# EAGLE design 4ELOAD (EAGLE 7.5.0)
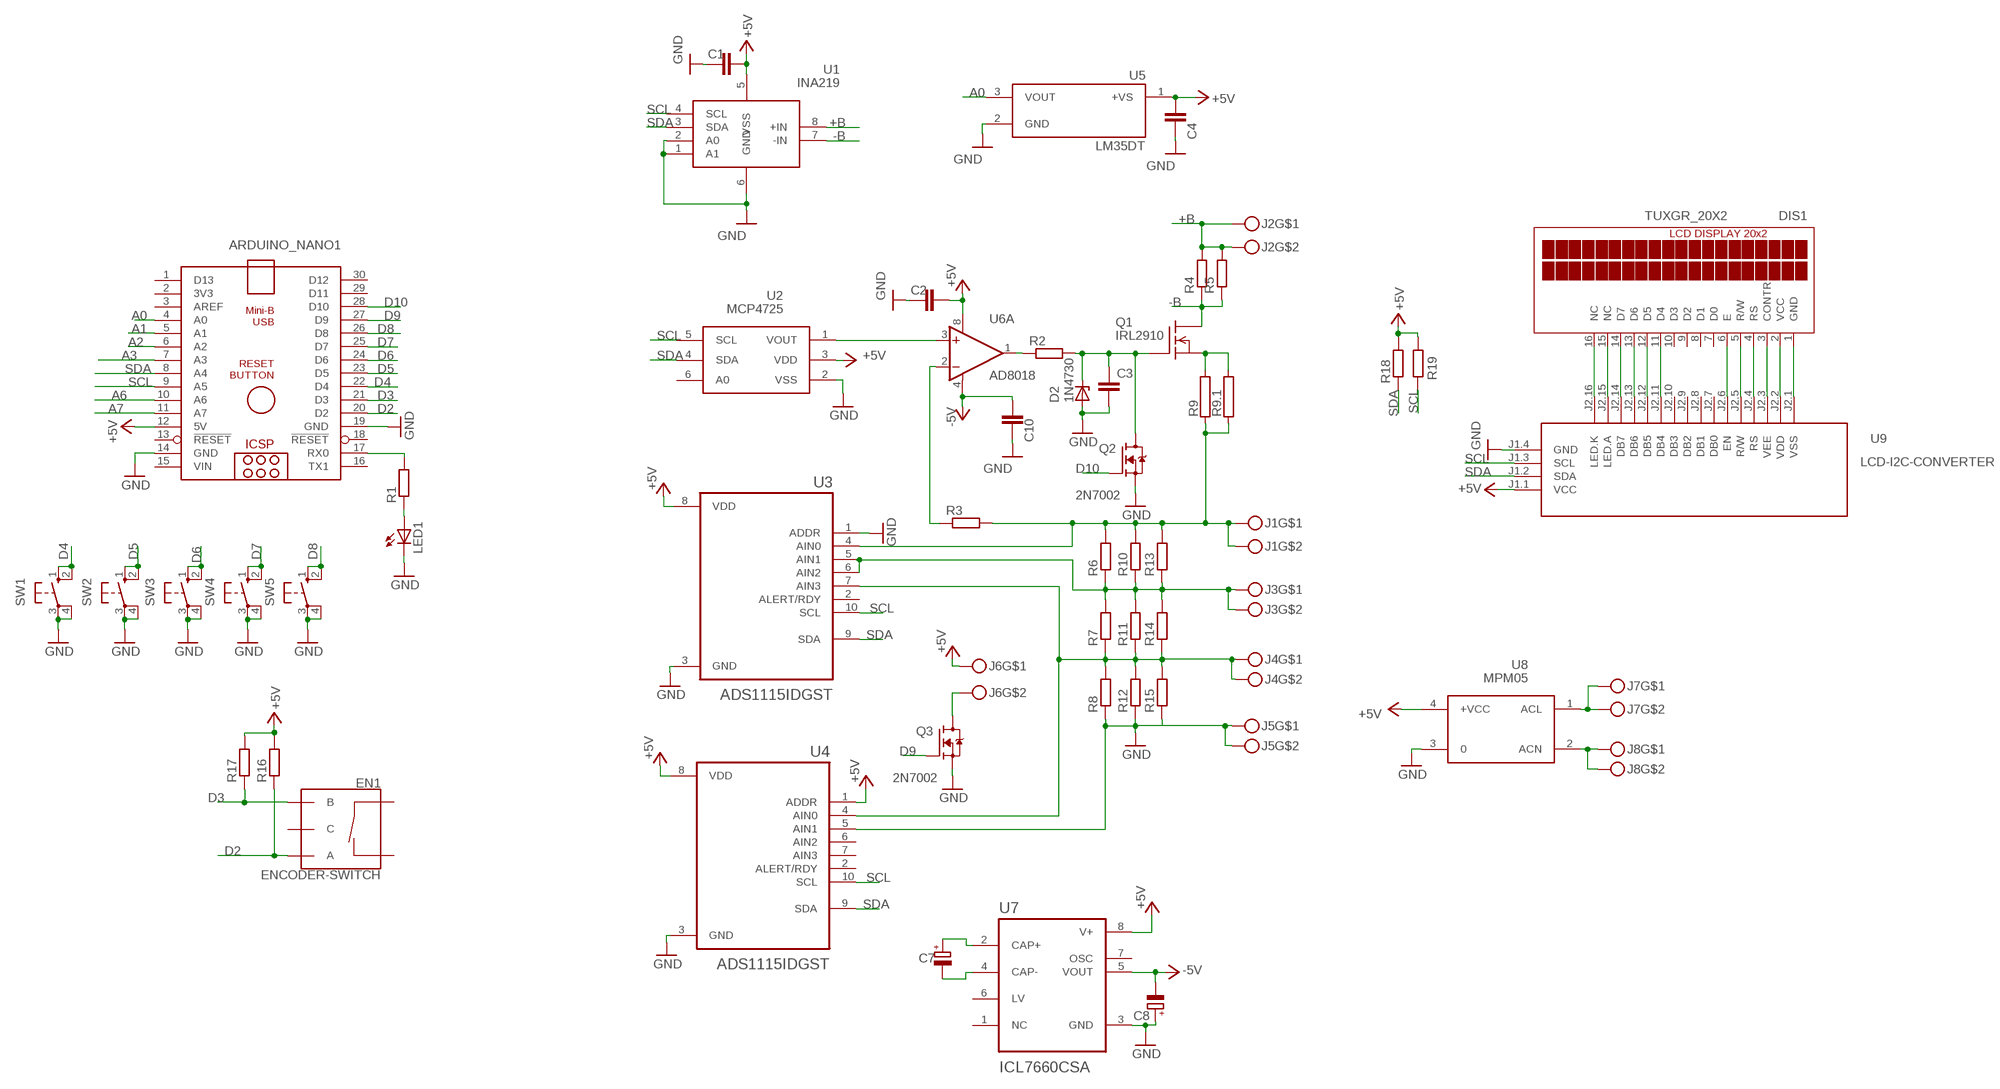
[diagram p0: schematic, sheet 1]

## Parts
ARDUINO_NANO1  ARDUINO_NANO  [ARDUINO_NANO]
C1  C-EUC1206  [C1206]
C2  C-EUC1206  [C1206]
C3  C-EUC1206  [C1206]
C4  C-EUC1206  [C1206]
C7  CPOL-EUSMCB  [SMC_B]
C8  CPOL-EUSMCB  [SMC_B]
C10  C-EUC1206  [C1206]
D2  1N4730  BZX85  [DO41Z10]
DIS1  TUXGR_20X2  [TUXGR_20X2]
EN1  ENCODER-SWITCH  [ROTARY_ENC_PLAIN]
J1  MKDSN1,5-2-5,08  [MKDSN1,5-2-5,08]
J2  MKDSN1,5-2-5,08  [MKDSN1,5-2-5,08]
J3  MKDSN1,5-2-5,08  [MKDSN1,5-2-5,08]
J4  MKDSN1,5-2-5,08  [MKDSN1,5-2-5,08]
J5  MKDSN1,5-2-5,08  [MKDSN1,5-2-5,08]
J6  MKDSN1,5-2-5,08  [MKDSN1,5-2-5,08]
J7  MKDSN1,5-2-5,08  [MKDSN1,5-2-5,08]
J8  MKDSN1,5-2-5,08  [MKDSN1,5-2-5,08]
LED1  LED5MM  [LED5MM]
Q1  IRL2910  BUZ21  [TO220]
Q2  2N7002  [SOT95P240X111-3N]
Q3  2N7002  [SOT95P240X111-3N]
R1  R-EU_R1206  [R1206]
R2  R-EU_R1206  [R1206]
R3  R-EU_R1206  [R1206]
R4  R-EU_R2512  [R2512]
R5  R-EU_R2512  [R2512]
R6  R-EU_R2512  [R2512]
R7  R-EU_R2512  [R2512]
R8  R-EU_R2512  [R2512]
R9  RCA5100  [CA5100]
R9.1  RCA5100  [CA5100]
R10  R-EU_R2512  [R2512]
R11  R-EU_R2512  [R2512]
R12  R-EU_R2512  [R2512]
R13  R-EU_R2512  [R2512]
R14  R-EU_R2512  [R2512]
R15  R-EU_R2512  [R2512]
R16  R-EU_R1206  [R1206]
R17  R-EU_R1206  [R1206]
R18  R-EU_R1206  [R1206]
R19  R-EU_R1206  [R1206]
SW1  10-XX  [B3F-10XX]
SW2  10-XX  [B3F-10XX]
SW3  10-XX  [B3F-10XX]
SW4  10-XX  [B3F-10XX]
SW5  10-XX  [B3F-10XX]
U1  INA219  [SO08]
U2  MCP4725  [SOT23-6]
U3  ADS1115IDGST  [SOP50P490X110-10N]
U4  ADS1115IDGST  [SOP50P490X110-10N]
U5  LM35DT  [TO254P1016X457X1955-3]
U6  AD8018  OPA2650U  [SO08]
U7  ICL7660CSA  [SOIC127P600X175-8N]
U8  MPM05  [MPM05]
U9  LCD-I2C-CONVERTER  [LCD-I2C-CONVERTER]

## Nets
+5V: ARDUINO_NANO1.12(5V) C1.1 C2.1 C4.1 DIS1.2(VCC) J6.1 R16.2 R17.2 R18.2 R19.2 U1.5(VSS) U2.3(VDD) U3.8(VDD) U4.1(ADDR) U4.8(VDD) U5.1(+VS) U6.8(A:V+) U7.8(V+) U8.4(+VCC) U9.J1.1(VCC) U9.J2.2(VDD)
+B: J2.1 J2.2 R4.2 R5.2 U1.8(+IN)
-5V: C8.- C10.1 U6.4(A:V-) U7.5(VOUT)
-B: Q1.2(D) R4.1 R5.1 U1.7(-IN)
A0: ARDUINO_NANO1.4(A0) U5.3(VOUT)
A1: ARDUINO_NANO1.5(A1)
A2: ARDUINO_NANO1.6(A2)
A3: ARDUINO_NANO1.7(A3)
A6: ARDUINO_NANO1.10(A6)
A7: ARDUINO_NANO1.11(A7)
D2: ARDUINO_NANO1.20(D2) EN1.A R16.1
D3: ARDUINO_NANO1.21(D3) EN1.B R17.1
D4: ARDUINO_NANO1.22(D4) SW1.1(S) SW1.2(S1)
D5: ARDUINO_NANO1.23(D5) SW2.1(S) SW2.2(S1)
D6: ARDUINO_NANO1.24(D6) SW3.1(S) SW3.2(S1)
D7: ARDUINO_NANO1.25(D7) SW4.1(S) SW4.2(S1)
D8: ARDUINO_NANO1.26(D8) SW5.1(S) SW5.2(S1)
D9: ARDUINO_NANO1.27(D9) Q3.1(G)
D10: ARDUINO_NANO1.28(D10) Q2.1(G)
GND: ARDUINO_NANO1.14(GND) ARDUINO_NANO1.19(GND) C1.2 C2.2 C3.2 C4.2 C8.+ C10.2 D2.A DIS1.1(GND) J5.1 J5.2 LED1.K(C) Q2.2(S) Q3.2(S) R8.1 R12.1 R15.1 SW1.3(P) SW1.4(P1) SW2.3(P) SW2.4(P1) SW3.3(P) SW3.4(P1) SW4.3(P) SW4.4(P1) SW5.3(P) SW5.4(P1) U1.1(A1) U1.2(A0) U1.6(GND) U2.2(VSS) U3.1(ADDR) U3.3(GND) U4.3(GND) U4.5(AIN1) U5.2(GND) U7.3(GND) U8.3 U9.J1.4(GND) U9.J2.1(VSS)
N$1: U2.1(VOUT) U6.3(A:+IN)
N$2: C3.1 D2.C Q1.1(G) Q2.3(D) R2.2
N$3: R2.1 U6.1(A:OUT)
N$4: Q1.3(S) R9.1.2 R9.2
N$5: R3.1 U6.2(A:-IN)
N$6: J1.1 J1.2 R3.2 R6.2 R9.1 R9.1.1 R10.2 R13.2 U3.4(AIN0)
N$7: ARDUINO_NANO1.17(RX0) R1.2
N$8: LED1.A R1.1
N$9: J3.1 J3.2 R6.1 R7.2 R10.1 R11.2 R13.1 R14.2 U3.5(AIN1) U3.6(AIN2)
N$10: J4.1 J4.2 R7.1 R8.2 R11.1 R12.2 R14.1 R15.2 U3.7(AIN3) U4.4(AIN0)
N$11: C7.+ U7.2(CAP+)
N$12: C7.- U7.4(CAP-)
N$13: J6.2 Q3.3(D)
N$15: J7.1 J7.2 U8.1(ACL)
N$16: J8.1 J8.2 U8.2(ACN)
N$31: DIS1.3(CONTR) U9.J2.3(VEE)
N$32: DIS1.4(RS) U9.J2.4(RS)
N$33: DIS1.5(R/W) U9.J2.5(R/W)
N$34: DIS1.6(E) U9.J2.6(EN)
N$35: DIS1.14(D7) U9.J2.14(DB7)
N$36: DIS1.13(D6) U9.J2.13(DB6)
N$37: DIS1.12(D5) U9.J2.12(DB5)
N$38: DIS1.11(D4) U9.J2.11(DB4)
N$39: DIS1.16(NC) U9.J2.16(LED.K)
N$40: DIS1.15(NC) U9.J2.15(LED.A)
SCL: ARDUINO_NANO1.9(A5) R19.1 U1.4(SCL) U2.5(SCL) U3.10(SCL) U4.10(SCL) U9.J1.3(SCL)
SDA: ARDUINO_NANO1.8(A4) R18.1 U1.3(SDA) U2.4(SDA) U3.9(SDA) U4.9(SDA) U9.J1.2(SDA)
Unconnected: ARDUINO_NANO1.1(D13) ARDUINO_NANO1.2(3V3) ARDUINO_NANO1.3(AREF) ARDUINO_NANO1.13(!RESET) ARDUINO_NANO1.16(TX1) ARDUINO_NANO1.18(!RESET) ARDUINO_NANO1.29(D11) ARDUINO_NANO1.30(D12) DIS1.7(D0) DIS1.8(D1) DIS1.9(D2) DIS1.10(D3) EN1.C EN1.SW+ EN1.SW- U2.6(A0) U3.2(ALERT/RDY) U4.2(ALERT/RDY) U4.6(AIN2) U4.7(AIN3) U6.5(B:+IN) U6.6(B:-IN) U6.7(B:OUT) U7.1(NC) U7.6(LV) U7.7(OSC) U9.J2.7(DB0) U9.J2.8(DB1) U9.J2.9(DB2) U9.J2.10(DB3)

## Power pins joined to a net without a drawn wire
VIN: ARDUINO_NANO1.15(VIN)

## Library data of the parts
ARDUINO_NANO1 = ArduinoNanoV30:ARDUINO_NANO: Arduino Nano V3.0 Overview: The Arduino Nano is a small, complete, and breadboard-friendly board based on the ATmega328 (Arduino Nano 3.x) or ATmega168 (Arduino Nano 2.x). It has more or less the same functionality of the Arduino Duemilanove, but in a different package. It lacks only a DC power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
C1-C4 C10 = rcl:C-EU: CAPACITOR, European symbol
C7 C8 = rcl:CPOL-EU: POLARIZED CAPACITOR, European symbol
D2 = diode:BZX85: Z DIODE
DIS1 = display-lcd:TUXGR_20X2: Tuxgraphics LCD display 20x2 characters reflective, without background light Source: tuxgr_20x2.pdf; OC_FARNELL: unknown; OC_NEWARK: unknown
EN1 = SparkFun-Switches:ENCODER-SWITCH: Rotary Encoder w/ Select Switch Encoders rotate similarly to potentiometers, but they’re different from potentiometers in that an encoder has full rotation without limits. They output gray code so that you can tell how much and in which direction the encoder has been turned. This encoder includes a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; SF_SKU: COM-09117
J1-J8 = con-phoenix-508:MKDSN1,5-2-5,08
LED1 = led:LED: LED
Q1 = transistor-fet:BUZ21: N-Channel Enhancement MOSFET 100V; 19A; 0,1Ohm
Q2 Q3 = 2N7002:2N7002: Check availability; AVAILABILITY: In Stock; CHECK_PRICES: https://www.snapeda.com/parts/2N7002/Onsemi/view-part/?ref=eda; DESCRIPTION: Mosfet Array 2 N-Channel (Dual) 60V 300mA 500mW Surface Mount PG-SOT363-6; MF: onsemi; MP: 2N7002; PACKAGE: SOT-23-3 ON Semiconductor; PRICE: None; SNAPEDA_LINK: https://www.snapeda.com/parts/2N7002/Onsemi/view-part/?ref=snap
R1-R8 R10-R19 = rcl:R-EU_: RESISTOR, European symbol
R9 R9.1 = resistor-power:R: Power Resitor; OC_FARNELL: unknown; OC_NEWARK: unknown
SW1-SW5 = switch-omron:10-XX: OMRON SWITCH; MPN: B3F-1000; OC_FARNELL: 176432; OC_NEWARK: 36M3542
U1 = burr-brown:INA219: Bidirectional Current/Power Monitor With I2C Interface
U2 = linear:MCP4725
U3 U4 = ADS1115IDGST:ADS1115IDGST: Check availability; AVAILABILITY: In Stock; CHECK_PRICES: https://www.snapeda.com/parts/ADS1115IDGST/Texas+Instruments/view-part/?ref=eda; DESCRIPTION: 16-bit, 860-SPS, 4-channel, delta-sigma ADC with PGA, oscillator, VREF, comparator and I2C; MF: Texas Instruments; MP: ADS1115IDGST; PACKAGE: VSSOP-10 Texas Instruments; PRICE: None; SNAPEDA_LINK: https://www.snapeda.com/parts/ADS1115IDGST/Texas+Instruments/view-part/?ref=snap
U5 = LM35DT-H:LM35DT: Check availability; AVAILABILITY: In Stock; CHECK_PRICES: https://www.snapeda.com/parts/LM35DT/Texas+Instruments/view-part/?ref=eda; DESCRIPTION: ±0.5°C 4V-30V, Temperature sensor with analog output 3-TO-220 0 to 100; MF: Texas Instruments; MP: LM35DT; PACKAGE: TO-220-3 Texas Instruments; PRICE: None; SNAPEDA_LINK: https://www.snapeda.com/parts/LM35DT/Texas+Instruments/view-part/?ref=snap
U6 = burr-brown:OPA2650: Dual Wideband, Low Power Voltage Feedback Operational Amplifier; MF: ALTERA CORPORATION; MPN: AD8056ARMZ; OC_FARNELL: 1424046; OC_NEWARK: 59K6306
U7 = ICL7660CSA:ICL7660CSA: Check availability; AVAILABILITY: In Stock; CHECK_PRICES: https://www.snapeda.com/parts/ICL7660CSA/Analog+Devices/view-part/?ref=eda; DESCRIPTION: Charge Pump Switching Regulator IC Positive or Negative Fixed -Vin, nVin, Vin/2 1 Output 20mA 8-SOIC (0.154, 3.90mm Width); MF: Analog Devices; MP: ICL7660CSA; PACKAGE: SOIC-8 Maxim; PRICE: None; SNAPEDA_LINK: https://www.snapeda.com/parts/ICL7660CSA/Analog+Devices/view-part/?ref=snap
U8 = acdc:MPM05: AC DC Converter 5W
U9 = diy-modules:LCD-I2C-CONVERTER: I2C Bus to 4-Bit Parallel LCD Interface with LED backlight driver

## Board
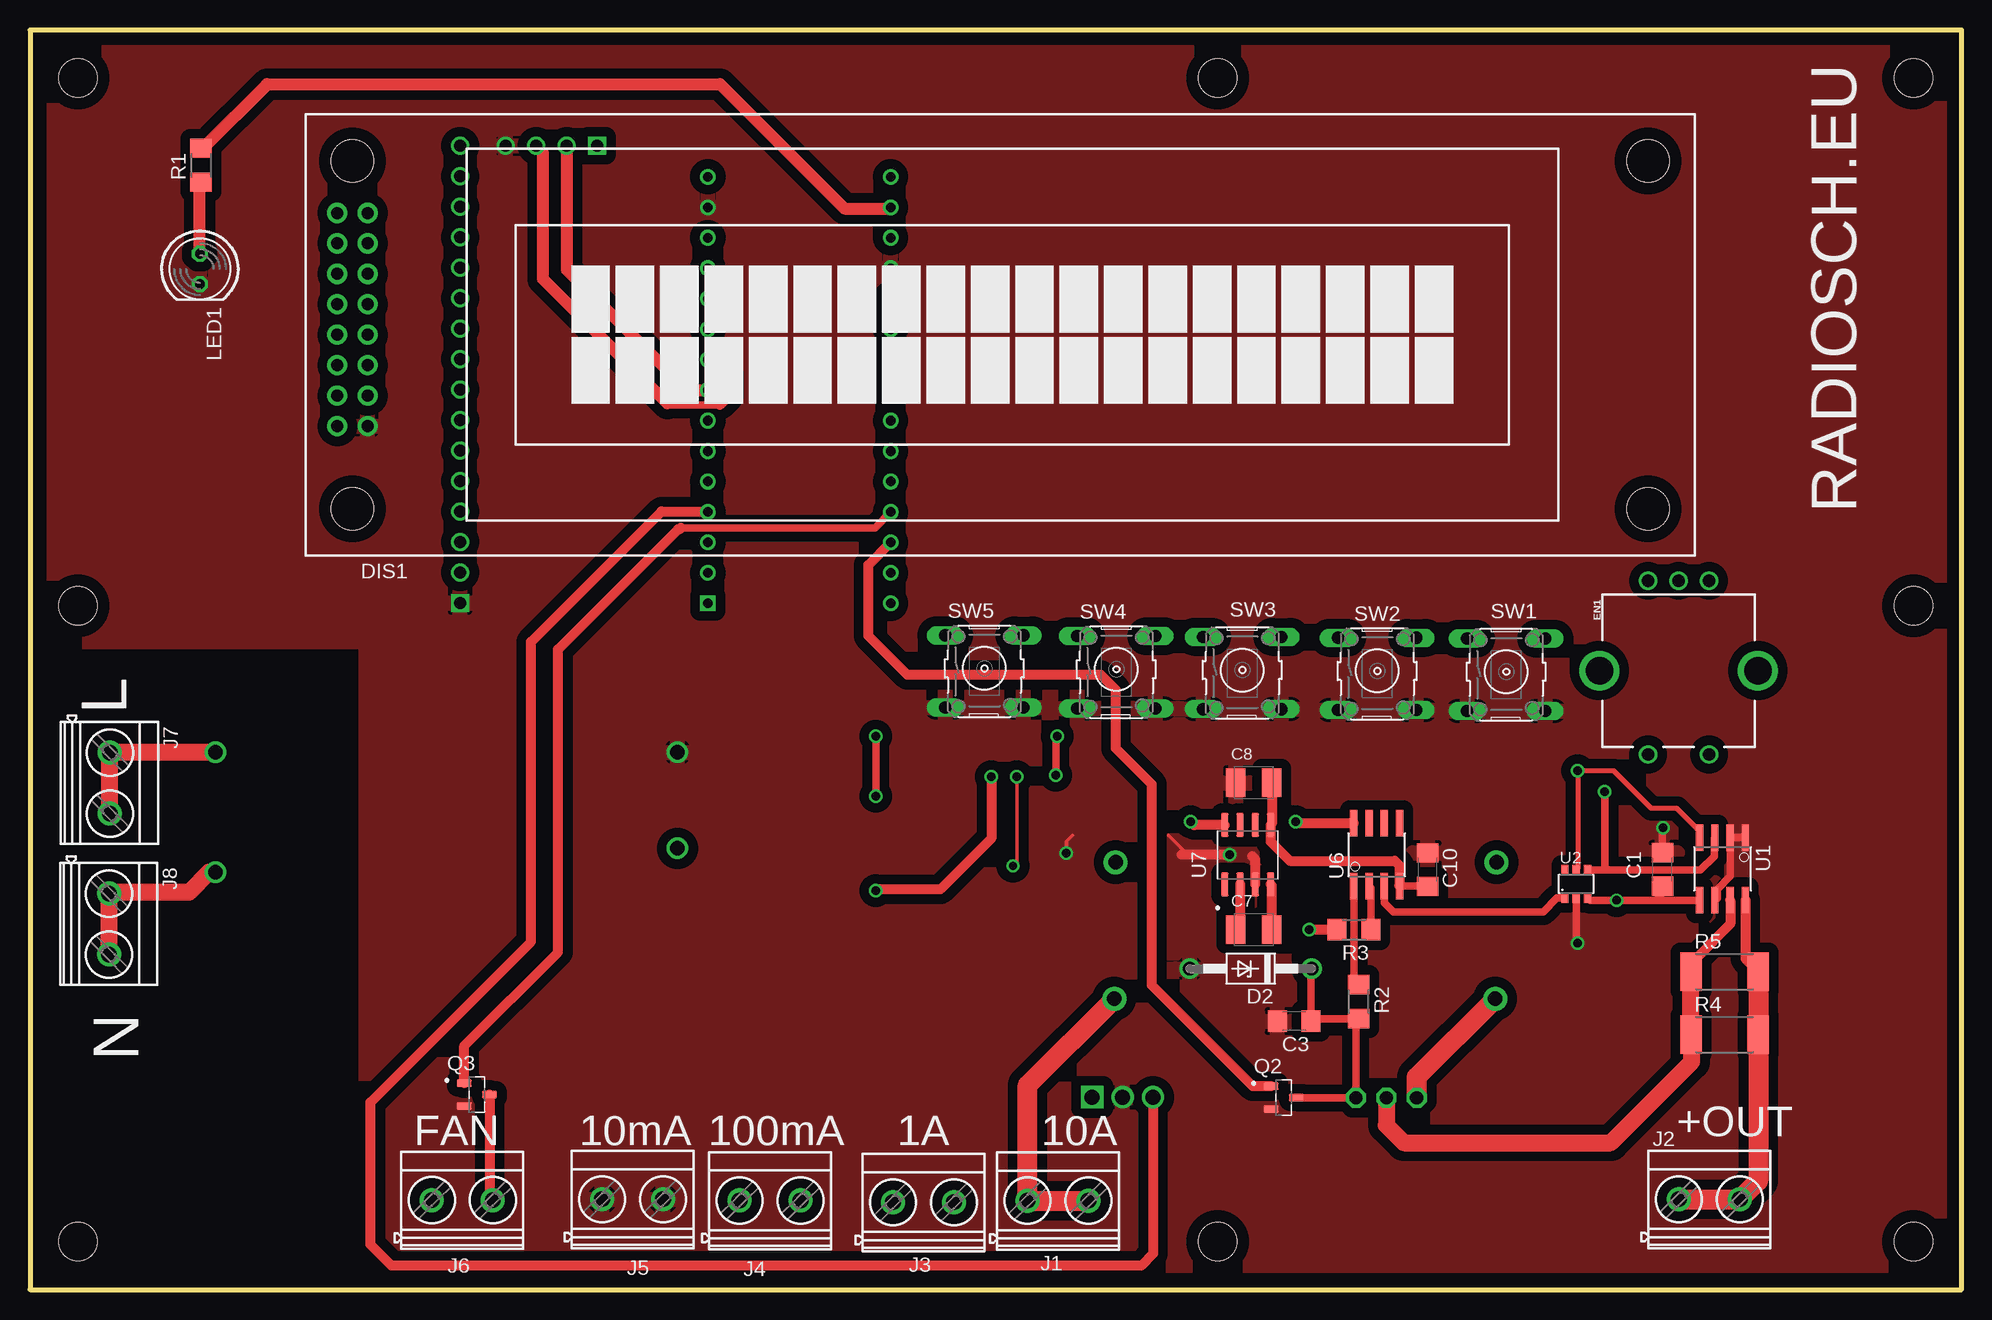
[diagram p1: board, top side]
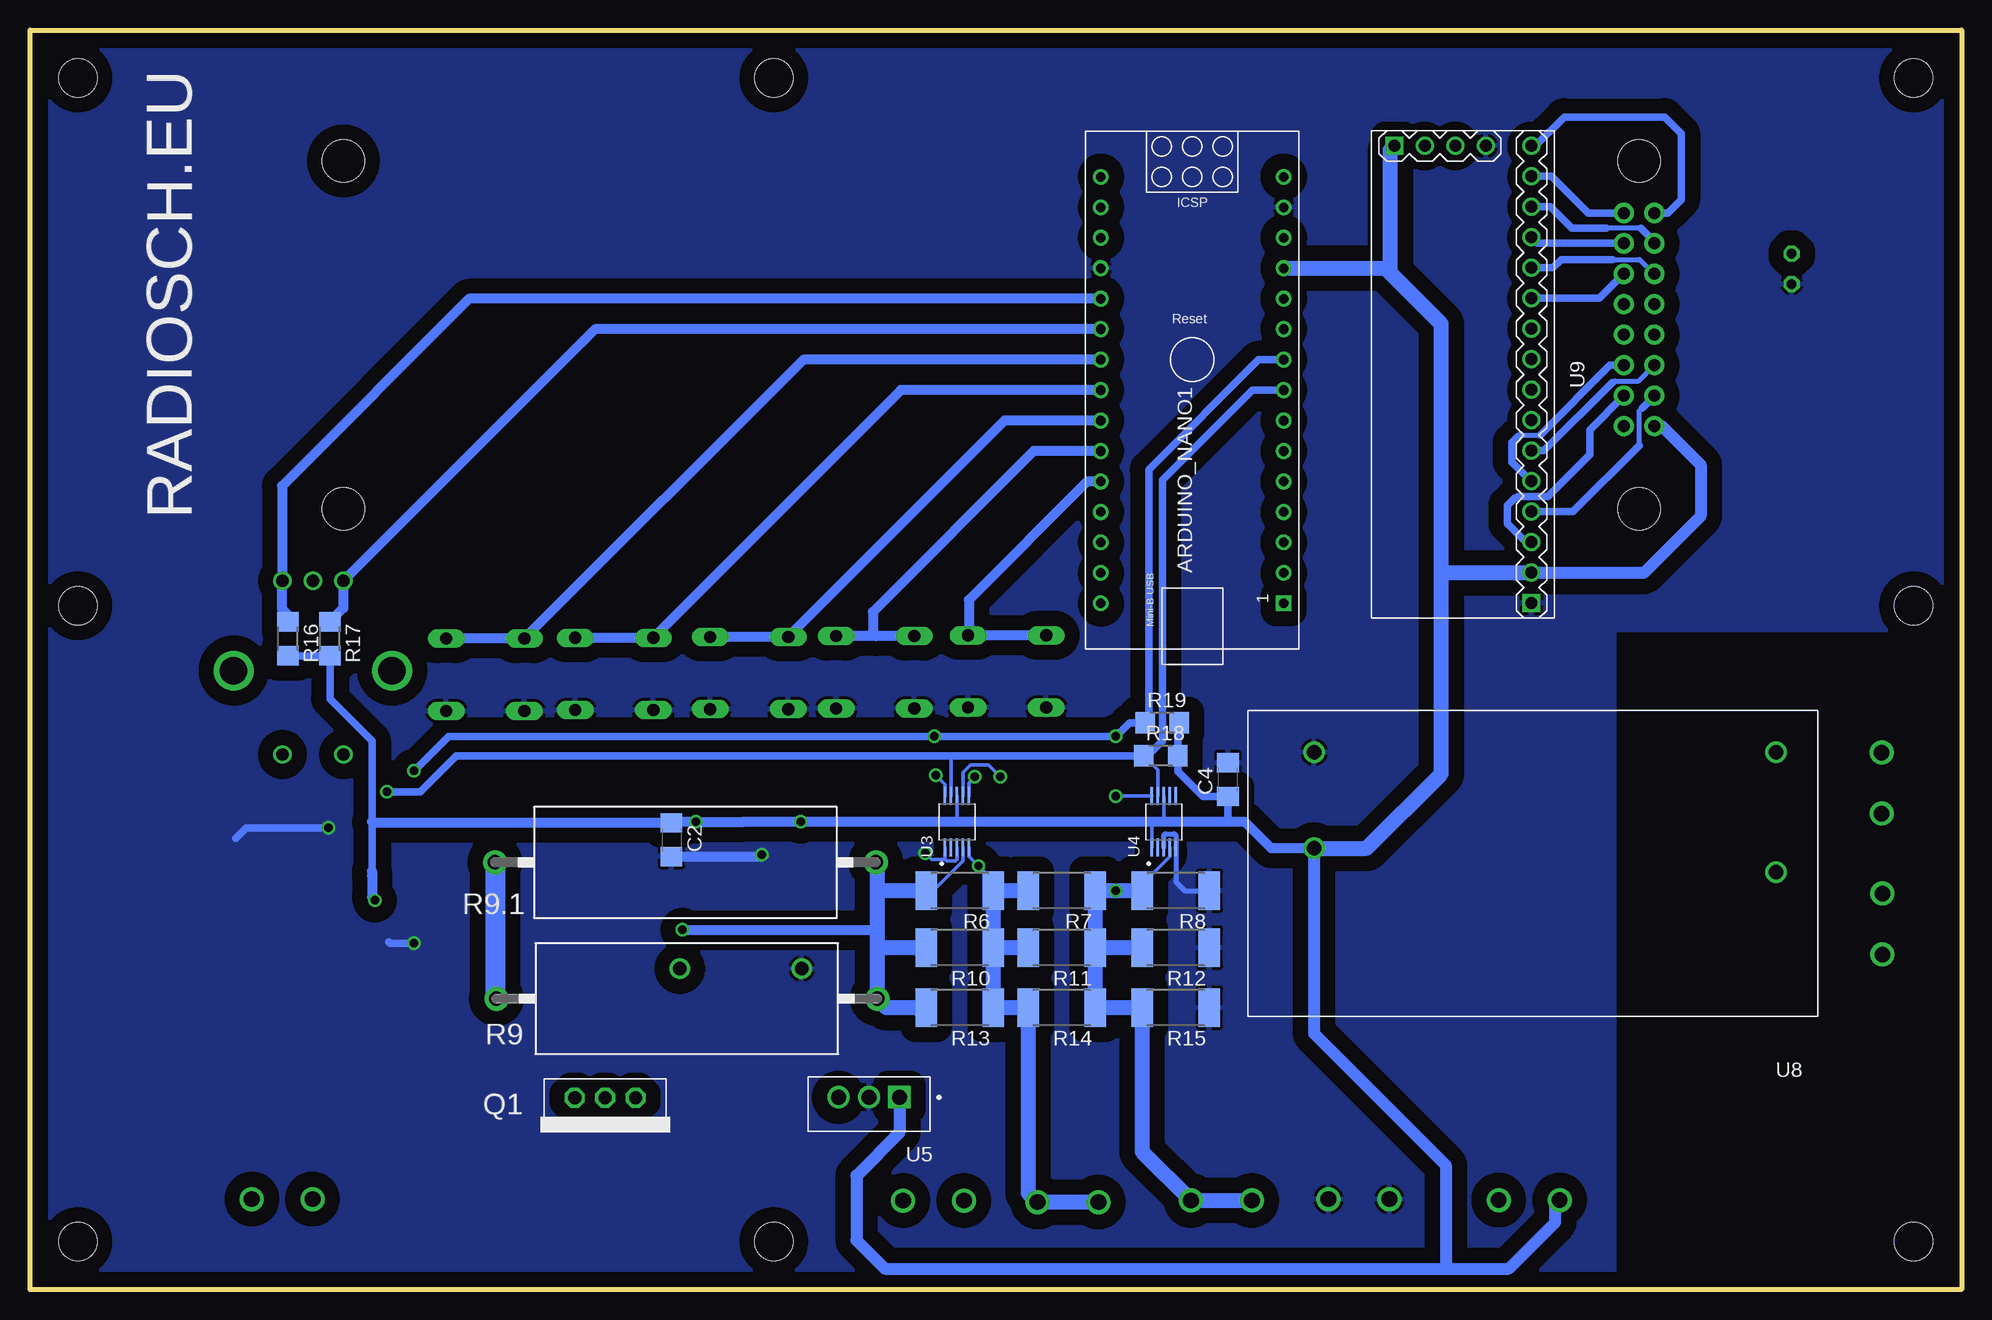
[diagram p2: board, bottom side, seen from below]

Size 161 x 105 mm. Coordinates in mm from the lower left corner, seen from the top.
Outline: 0,0 161,0 161,105 0,105 0,0
Copper layers (1*16): Top 0.035mm / dielectric 1.5mm / Bottom 0.035mm
Design rules "default *": minimum track width 10mil, minimum drill 24mil, track to track 4mil, track to pad 4mil, pad to pad 4mil, via to via 8mil, smd to smd 4mil, copper to edge 40mil, drill to drill 8mil, minimum pad ring 10mil, minimum via ring 8mil, stop-mask expansion 4mil, vias tented up to drill 0mil, thermal gap 10mil
Holes 3.2 mm at 4,4 99,4 157,4 4,57 157,57 157,101 99,101 4,101

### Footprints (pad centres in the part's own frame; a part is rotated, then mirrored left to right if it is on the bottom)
ARDUINO_NANO = drill 0.8 square: 1 -20.32,-7.62 | drill 0.8: 2 -17.78,-7.62; 3 -15.24,-7.62; 4 -12.7,-7.62; 5 -10.16,-7.62; 6 -7.62,-7.62; 7 -5.08,-7.62; 8 -2.54,-7.62; 9 0,-7.62; 10 2.54,-7.62; 11 5.08,-7.62; 12 7.62,-7.62; 13 10.16,-7.62; 14 12.7,-7.62; 15 15.24,-7.62; 16 15.24,7.62; 17 12.7,7.62; 18 10.16,7.62; 19 7.62,7.62; 20 5.08,7.62; 21 2.54,7.62; 22 0,7.62; 23 -2.54,7.62; 24 -5.08,7.62; 25 -7.62,7.62; 26 -10.16,7.62; 27 -12.7,7.62; 28 -15.24,7.62; 29 -17.78,7.62; 30 -20.32,7.62
C1206 = smd 1.6 x 1.8: 1 -1.4,0; 2 1.4,0
SMC_B = smd 1.6 x 2.4: + -1.5,0; - 1.5,0
DO41Z10 = drill 1.118: A 5.08,0; C -5.08,0
TUXGR_20X2 = drill 1 pad 1.676: 1 -52.73,-7.62; 2 -55.27,-7.62; 3 -52.73,-5.08; 4 -55.27,-5.08; 5 -52.73,-2.54; 6 -55.27,-2.54; 7 -52.73,0; 8 -55.27,0; 9 -52.73,2.54; 10 -55.27,2.54; 11 -52.73,5.08; 12 -55.27,5.08; 13 -52.73,7.62; 14 -55.27,7.62; 15 -52.73,10.16; 16 -55.27,10.16 | hole 3.5: -54,-14.5; 54,-14.5; -54,14.5; 54,14.5
ROTARY_ENC_PLAIN = drill 1.016: A 7.493,-2.54; B 7.493,2.54; C 7.493,0; SW+ -6.985,2.54; SW- -6.985,-2.54 | drill 2.286: P$3 0,6.604; P$4 0,-6.604
MKDSN1,5-2-5,08 = drill 1.3 pad 2: 1 -2.561,0.025; 2 2.519,0.025
LED5MM = drill 0.813 octagon: A -1.27,0; K 1.27,0
TO220 = drill 1.118 octagon: 1 -2.54,0; 2 0,0; 3 2.54,0
SOT95P240X111-3N = smd 1.23 x 0.6: 1 -1.06,0.95; 2 -1.06,-0.95; 3 1.06,0
R1206 = smd 1.6 x 1.803: 1 -1.422,0; 2 1.422,0
R2512 = smd 1.8 x 3.2: 1 -2.8,0; 2 2.8,0
CA5100 = drill 1.2 pad 2: 1 -15.875,0; 2 15.875,0
B3F-10XX = drill 1.016 long: 1 -3.251,2.761; 2 3.251,2.761; 3 -3.251,-3.261; 4 3.251,-3.261
SO08 = smd 0.61 x 2.21: 1 -1.905,-2.616; 2 -0.635,-2.616; 3 0.635,-2.616; 4 1.905,-2.616; 5 1.905,2.616; 6 0.635,2.616; 7 -0.635,2.616; 8 -1.905,2.616
SOT23-6 = smd 0.6 x 0.9: 1 -0.95,-1.15; 2 0,-1.15; 3 0.95,-1.15; 4 0.95,1.15; 5 0,1.15; 6 -0.95,1.15
SOP50P490X110-10N = smd 1.47 x 0.28: 1 -2.15,1; 2 -2.15,0.5; 3 -2.15,0; 4 -2.15,-0.5; 5 -2.15,-1; 6 2.15,-1; 7 2.15,-0.5; 8 2.15,0; 9 2.15,0.5; 10 2.15,1
TO254P1016X457X1955-3 = drill 1.24 square: 1 -2.54,-0.573 | drill 1.24: 2 0,-0.573; 3 2.54,-0.573
SOIC127P600X175-8N = smd 1.97 x 0.59: 1 -2.475,1.905; 2 -2.475,0.635; 3 -2.475,-0.635; 4 -2.475,-1.905; 5 2.475,-1.905; 6 2.475,-0.635; 7 2.475,0.635; 8 2.475,1.905
MPM05 = drill 1.2: 1 3.5,-22; 2 3.5,-12; 3 42,-22; 4 42,-14
LCD-I2C-CONVERTER = drill 1 square: J1.1 -19.05,-5.08; J2.1 19.05,6.35 | drill 1: J1.2 -19.05,-2.54; J1.3 -19.05,0; J1.4 -19.05,2.54; J2.2 16.51,6.35; J2.3 13.97,6.35; J2.4 11.43,6.35; J2.5 8.89,6.35; J2.6 6.35,6.35; J2.7 3.81,6.35; J2.8 1.27,6.35; J2.9 -1.27,6.35; J2.10 -3.81,6.35; J2.11 -6.35,6.35; J2.12 -8.89,6.35; J2.13 -11.43,6.35; J2.14 -13.97,6.35; J2.15 -16.51,6.35; J2.16 -19.05,6.35

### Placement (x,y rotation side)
ARDUINO_NANO1  64.12,77.52 90 bottom
C1  136.07,35.02 90 top
C2  107.53,37.49 270 bottom
C3  105.38,22.38 180 top
C4  61.15,42.51 90 bottom
C7  102,30 0 top
C8  102,42.25 0 top
C10  116.5,35 90 top
D2  101.75,26.75 180 top
DIS1  80.88,79.59 0 top
EN1  137.42,51.59 90 top
J1  85.71,7.38 0 top
J2  140,7.5 0 top
J3  74.5,7.25 0 top
J4  61.71,7.4 0 top
J5  50.25,7.5 0 top
J6  36.05,7.43 0 top
J7  6.63,42.2 270 top
J8  6.56,30.45 270 top
LED1  14.16,85.08 270 top
Q1  113.06,15.98 180 bottom
Q2  104.5,16 0 top
Q3  37.25,16.25 0 top
R1  14.26,93.73 90 top
R2  110.75,24 270 top
R3  110.35,30 180 top
R4  141.25,21.25 0 top
R5  141.25,26.5 0 top
R6  83.5,33.25 180 bottom
R7  75,33.25 180 bottom
R8  65.5,33.25 180 bottom
R9  106.25,24.25 180 bottom
R9.1  106.37,35.61 180 bottom
R10  83.5,28.5 180 bottom
R11  75,28.5 180 bottom
R12  65.5,28.5 180 bottom
R13  83.5,23.5 180 bottom
R14  75,23.5 180 bottom
R15  65.5,23.5 180 bottom
R16  139.5,54.25 270 bottom
R17  136,54.25 270 bottom
R18  66.75,44.5 0 bottom
R19  66.62,47.25 0 bottom
SW1  123.05,51.5 0 top
SW2  112.3,51.57 0 top
SW3  101.05,51.64 0 top
SW4  90.55,51.71 0 top
SW5  79.55,51.78 0 top
U1  141.08,35.06 180 top
U2  128.88,33.81 0 top
U3  83.75,39 90 bottom
U4  66.5,39 90 bottom
U5  91.07,15.46 180 bottom
U6  112.25,36.25 0 top
U7  101.5,36.25 90 top
U8  11.97,22.78 180 bottom
U9  42.2,76.29 270 bottom

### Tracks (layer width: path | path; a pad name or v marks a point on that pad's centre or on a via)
+5V  (via drill 0.7)
  Top 0.61: U1.5 135.5,32.44 | 135.5,32.44 v132.25,32.44 130.05,32.44 U2.3 | C1.1 136.07,33.01 135.5,32.44
  Top 0.813: U7.8 97.03,38.73 v96.75,39 | U6.8 105.63,38.87 v105.5,39
  Bottom 0.305: U4.8 66.5,39.12 66.62,39 | U4.1 67.5,38.88 67.38,39 | U3.8 83.75,39.25 84,39
  Bottom 0.61: 61.38,39 61.15,39.23 C4.1 61.16,41.12 63.25,41.12 65.33,43.2 R18.2 65.33,47.12 R19.2 | R16.2 R17.2 136,49.25 132.5,45.75 132.5,39 132.5,34.5
  Bottom 0.813: U8.4 57.53,36.78 59.75,39 61.38,39 66.62,39 67.38,39 84,39 v96.75,39 101.5,39 v105.5,39 107.42,39 C2.1 132.39,38.89 132.5,39 | 132.5,34.88 132.5,34.5 132.5,32.69 v132.25,32.44
  Bottom 1.016: U5.1 88.53,13.1 92.12,9.5 92.12,4.12 89.75,1.75 42.75,1.75 | 42.75,1.75 37.75,1.75 33.88,5.62 33.88,7.07 J6.1 | U8.4 53.97,21.34 43,10.38 43,2 42.75,1.75 | DIS1.2 24.97,71.97 21.75,68.75 21.75,64.5 26.5,59.75 35.82,59.75 U9.J2.2
  Bottom 1.27: U8.4 49.59,36.78 43.38,43 43.38,59.5 | U9.J2.2 35.88,59.75 43.12,59.75 43.38,59.5 | 43.38,59.5 43.38,80.5 47.62,84.75 | 47.62,84.75 47.62,95 U9.J1.1 | ARDUINO_NANO1.12 48.02,85.14 47.62,84.75
+B
  Top 0.813: U1.8 142.99,27.57 R5.2
  Top 1.676: R5.2 R4.2 144.05,9.06 J2.2 J2.1
-5V
  Top 0.61: U6.4 116.47,33.63 C10.1
  Top 0.813: U6.4 114.12,33.66 114.12,35.38 113.75,35.75 105,35.75 103.41,37.34 U7.5 103.5,38.82 C8.-
-B
  Top 0.813: U1.7 141.72,30.46 138.88,27.62 138.88,26.93 R5.1
  Top 1.422: Q1.2 113.06,13.69 114.5,12.25 131.75,12.25 138.5,19 138.5,21.2 R4.1 R5.1
A0
  Top 0.813: U5.3 93.61,2.98 92.62,2 30.12,2 28.38,3.75 28.38,15.62 41.75,29 41.75,54 52.62,64.88 56.45,64.88 ARDUINO_NANO1.4
D2
  Bottom 0.813: R16.1 139.5,56.25 140,56.75 140,59.04 EN1.A 140,59.12 140,67 124.4,82.6 ARDUINO_NANO1.20
D3
  Bottom 0.813: R17.1 134.88,56.79 EN1.B 113.9,80.06 ARDUINO_NANO1.21
D4
  Bottom 0.813: ARDUINO_NANO1.22 96.54,77.52 SW1.1 SW1.2
D5
  Bottom 0.813: ARDUINO_NANO1.23 88.4,74.98 SW2.1 SW2.2
D6
  Bottom 0.813: ARDUINO_NANO1.24 79.76,72.44 SW3.1 SW3.2
D7
  Bottom 0.813: SW4.1 90.5,54.47 | 90.5,54.47 SW4.2 | ARDUINO_NANO1.25 77.35,69.9 90.75,56.5 90.75,54.72 90.5,54.47
D8
  Bottom 0.813: SW5.1 SW5.2 82.75,54.59 82.75,57.5 72.89,67.36 ARDUINO_NANO1.26
D9
  Top 0.61: 54.25,63.5 70.42,63.5 ARDUINO_NANO1.27
  Top 0.813: Q3.1 36.19,20.31 44,28.12 44,53.38 54,63.38 54.12,63.38 54.25,63.5
D10
  Top 0.813: Q2.1 101.92,16.95 93.5,25.38 93.5,42.12 90.5,45.12 90.5,50 89.25,51.25 73.12,51.25 69.88,54.5 69.88,60.41 ARDUINO_NANO1.28
GND  (via drill 0.7)
  Top 0.305: v86.38,36.38 86.38,37.38 86.88,37.88 | 94.88,37.88 96.5,36.25
  Top 0.61: U2.2 128.88,29 v129,28.88 | U1.1 U1.2 141.72,34.47 140.62,33.38 140.62,32.62 U1.6 | C1.2 136.07,38.45 v136.12,38.5
  Top 0.813: U7.3 102.14,35.86 101.88,36.12 | v100,36.25 96.5,36.25 96,36.25
  Bottom 0.305: U3.3 83.75,35.88 83.88,35.75 84.62,35.75 84.75,35.88 | 84.75,35.88 U3.1 | 84.75,35.88 85.88,35.88 v86.38,36.38
  Bottom 0.406: R8.1 64.75,33.25 65.5,34 U4.5 65.5,37.88 65.62,38 66.38,38 66.5,37.88 U4.3
  Bottom 0.61: v129,28.88 131,28.88 131.12,29 | v136.12,38.5 143,38.5 143.88,37.62
  Bottom 0.813: C2.2 100.16,36.09 v100,36.25
  pour Bottom (isolate 1.27): 1,104 1,55 29,55 29,1 160,1 160,103 160,104
  pour Top (isolate 0.813): 2,104 160,104 160,2 28,2 28,54 2,54
N$1
  Top 0.61: U2.1 127.28,32.66 126.12,31.5 113.62,31.5 112.88,32.25 112.88,33.64 | 112.88,34.12 112.88,33.64 | 112.88,33.64 U6.3
N$2
  Top 0.61: Q2.3 110.5,16 Q1.1 110.52,22.35 R2.2 106.98,22.58 C3.1 106.78,26.7 D2.C
N$3
  Top 0.61: U6.1 110.34,25.83 R2.1
N$4
  Top 1.676: Q1.3 115.6,17.73 R9.2
  Bottom 1.676: R9.1.2 122.25,24.37 R9.2
N$5
  Top 0.61: R3.1 111.77,33.48 U6.2
N$6  (via drill 0.7)
  Top 0.813: R3.2 v106.62,30
  Top 1.676: R9.1 83.15,17.02 J1.1 J1.2
  Bottom 0.305: U3.4 83.25,35.75 85.38,33.62 85.92,33.62 R6.2
  Bottom 0.813: v106.62,30 90.62,30 90.38,29.75
  Bottom 1.27: 90.38,28.38 R9.1 89.62,23.5 R13.2 | 90.38,28.38 90.38,29.75 90.38,33.25 | 90.38,33.25 90.38,35.49 R9.1.1 | R10.2 90.25,28.5 90.38,28.38 | R6.2 90.38,33.25
N$7
  Top 1.016: R1.2 14.4,95.15 19.75,100.5 57.5,100.5 67.88,90.12 71.65,90.12 ARDUINO_NANO1.17
N$8
  Top 1.016: LED1.A 14.16,92.21 R1.1
N$9  (via drill 0.7)
  Top 0.305: v82.25,42.75 82.25,35.62 v81.94,35.31
  Bottom 0.305: U3.5 82.75,36.12 v81.94,35.31 79.88,33.25 | U3.6 82.75,42.25 v82.25,42.75
  Bottom 1.27: R7.2 79.88,33.25 R6.1 R10.1 | R11.2 R10.1 | R10.1 R13.1 R14.2 77.8,8.06 J3.2 J3.1
N$10  (via drill 0.7)
  Top 0.813: v80.12,42.75 80.12,37.62 75.88,33.38 70.62,33.38 v70.5,33.25
  Bottom 0.305: U4.4 66,36.12 68,34.12 68,33.55 R8.2 | U3.7 83.25,43.12 82.62,43.75 81.12,43.75 v80.12,42.75
  Bottom 1.27: R8.2 69.12,33.25 v70.5,33.25 R7.1 R11.1 | R12.2 R11.1 | R11.1 R14.1 R15.2 68.3,11.5 J4.2 J4.1
N$11
  Top 0.813: U7.2 100.86,30.36 C7.+
N$12
  Top 0.813: C7.- 103.5,33.68 U7.4
N$13
  Top 0.813: Q3.3 38.31,7.71 J6.2
N$15
  Top 1.422: U8.1 7.16,44.78 7.12,44.75 J7.1 J7.2
N$16
  Top 1.422: U8.2 14.9,34.78 13.25,33.12 6.7,33.12 J8.1 J8.2
N$31
  Bottom 0.61: U9.J2.3 36.32,62.32 37.88,63.88 37.88,65.38 37.25,66 37.12,66 37,66.12 34.5,66.12 31,69.62 31,71.66 DIS1.3
N$32
  Bottom 0.406: 26.88,70.38 26.88,73.25 26.62,73.5
  Bottom 0.61: U9.J2.4 32.39,64.86 26.88,70.38 | 26.62,73.5 DIS1.4
N$33
  Bottom 0.406: 36.75,71.25 35.12,71.25
  Bottom 0.61: U9.J2.5 35.9,67.4 37.5,69 37.5,70.62 37,71.12 36.88,71.12 36.75,71.25 | DIS1.5 29.32,77.05 35.12,71.25
N$34
  Bottom 0.406: 29.12,75.62 29,75.62 28.88,75.75 26.91,75.75 DIS1.6
  Bottom 0.61: U9.J2.6 34.81,69.94 29.12,75.62
N$35
  Bottom 0.406: 26.75,88.5 29.62,88.5
  Bottom 0.61: U9.J2.14 34.26,90.26 32.5,88.5 29.62,88.5 | DIS1.14 25.61,87.36 26.75,88.5
N$36
  Bottom 0.61: DIS1.13 35.34,87.21 U9.J2.13
N$37
  Bottom 0.406: 29.12,85.88 26.81,85.88 DIS1.12
  Bottom 0.61: U9.J2.12 34.07,85.18 33.38,85.88 29.12,85.88
N$38
  Bottom 0.61: U9.J2.11 30.18,82.64 DIS1.11
N$39
  Bottom 0.61: U9.J2.16 35.53,95.34 33.12,97.75 24.75,97.75 23.38,96.38 23.38,90.88 24.5,89.75 DIS1.16
N$40
  Bottom 0.61: U9.J2.15 34.17,92.8 31.12,89.75 DIS1.15
SCL  (via drill 0.7)
  Top 0.305: 85.5,46 v85.62,46.12
  Top 0.406: U2.5 129,35.08 v129,43.25 132,43.25 135.12,40.12 137.25,40.12 139.18,38.2 U1.4
  Top 0.61: v70.5,41.12 v70.5,46.12 | v85.5,42.88 85.5,46 | 57.5,73.75 53.25,73.75 53.12,73.88
  Top 0.813: ARDUINO_NANO1.9 57.1,77.52 58.25,76.38 58.25,74.5 57.5,73.75
  Top 1.016: 53.12,73.88 42.75,84.25 42.75,94.79 U9.J1.3
  Bottom 0.305: U4.10 70.47,41.15 v70.5,41.12 | U3.10 84.75,42.12 v85.5,42.88
  Bottom 0.61: ARDUINO_NANO1.9 58.6,77.52 67.75,68.38 67.75,47.55 R19.1 69.38,47.25 v70.5,46.12 v85.62,46.12 126.12,46.12 v129,43.25
SDA  (via drill 0.7)
  Top 0.61: U2.4 131.5,34.96 | 131.5,34.96 139.21,34.96 140.38,36.12 140.38,37.61 U1.3 | v131.25,41.5 131.25,35.21 131.5,34.96
  Top 1.016: U9.J1.2 44.74,85.01 54.75,75 56.48,75 ARDUINO_NANO1.8
  Bottom 0.305: U4.9 67,43.33 R18.1 | U3.9 84.25,44.38 84.38,44.5
  Bottom 0.61: ARDUINO_NANO1.8 56.52,75 59.12,75 66.62,67.5 66.62,45.75 67.88,44.5 R18.1 84.38,44.5 125.5,44.5 128.5,41.5 v131.25,41.5

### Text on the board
tPlace: RADIOSCH.EU | L | N | +OUT | FAN | 10mA | 100mA | 1A | 10A
bPlace: RADIOSCH.EU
